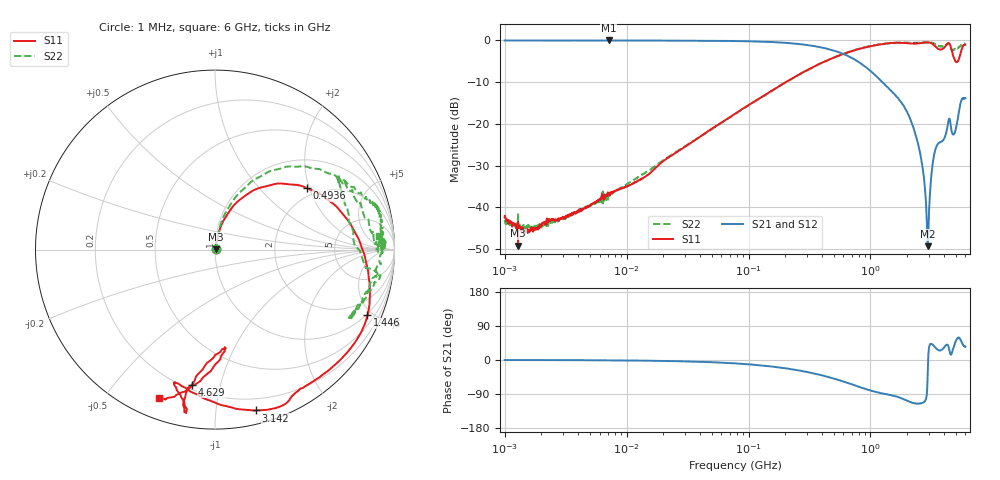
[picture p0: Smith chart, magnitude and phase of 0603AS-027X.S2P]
!s-Parameter Generated by FASTRON Sdn. Bhd.
!FASTRON P/N : 0603AS-027X
!Keysight Technologies: E5071C_MY46733604_B.14.02
!Date: Thu Nov 23 10:44:12 2023
!Version  :Rev01  Thu Nov 23 10:44:12 2023
!Data & Calibration Information:
!Freq  S11:SOLT2(ON)  S21:SOLT2(ON)  S12:SOLT2(ON)  S22:SOLT2(ON)
!PortZ  Port1:50+j0  Port2:50+j0
!When reading reference impedance value at option line is always used.
! Remarks : This data is being provided solely for informational purposes.
# Hz S dB R 50
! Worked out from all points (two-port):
!   1601 points, 1 MHz to 6 GHz, reference 50 ohm
!   highest |S21| = -0.04 dB at 7.15 MHz (marker M1); lowest = -49.3 dB at 2.951 GHz (marker M2)
!   |S21| within 3 dB of the highest: start of sweep to 570.2 MHz
!   lowest |S11| = -49.2 dB at 1.288 MHz (marker M3), VSWR 1.01, Z = 50.3 + j0.133 ohm
!   |S11| at or under -10 dB: start of sweep to 202.4 MHz
!   |S22| runs from -46.1 to -0.4 dB; largest |S21 - S12| = 0.0073
!   S11 on the Smith chart (normalised r, x): 1 MHz: 1.01, +0.01; 493.6 MHz: 1.74, +1.92; 1.446 GHz: 0.92, -4.68; 3.142 GHz: 0.10, -1.28; 4.629 GHz: 0.23, -0.82; 6 GHz: 0.09, -0.69
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1000000  -42.36 23.6  -0.04 -0.1  -0.05 -0.1  -43.05 22.6
1287650  -49.17 22.3  -0.05 -0.2  -0.02 -0.2  -41.46 12.8
4277066  -40.78 59.4  -0.06 -0.5  -0.05 -0.5  -40.67 59.7
7149933  -36.56 65.0  -0.04 -0.9  -0.06 -0.9  -37.04 74.5
1.823719e7  -29.93 77.7  -0.06 -2.2  -0.07 -2.2  -29.53 76.0
7.757876e7  -17.60 75.9  -0.17 -8.9  -0.18 -8.9  -17.66 77.6
3.307917e8  -6.56 49.6  -1.29 -34.3  -1.29 -34.3  -6.62 59.1
4.935518e8  -4.22 33.9  -2.41 -48.3  -2.41 -48.3  -4.21 48.8
8.659894e8  -1.84 2.7  -5.91 -74.0  -5.91 -74.1  -1.75 28.2
1.414819e9  -0.70 -22.3  -11.58 -92.0  -11.59 -92.0  -0.70 15.0
1.44567e9  -0.68 -23.3  -11.87 -92.2  -11.87 -92.2  -0.66 16.0
2.350488e9  -0.80 -59.2  -22.71 -114.6  -22.70 -114.5  -0.67 2.0
2.658144e9  -0.61 -63.5  -29.90 -113.5  -29.90 -113.4  -0.62 0.9
2.951149e9  -0.48 -68.2  -49.31 -27.5  -49.24 -27.3  -0.56 1.7
3.024401e9  -0.52 -70.6  -40.66 34.2  -40.63 34.1  -0.56 2.7
3.141603e9  -0.68 -75.7  -32.89 42.5  -32.87 42.4  -0.65 -0.9
3.42197e9  -1.55 -93.2  -25.92 31.8  -25.91 31.7  -1.07 -12.6
3.867453e9  -2.15 -106.8  -24.16 27.9  -24.18 27.8  -1.40 -26.1
4.312935e9  -0.73 -100.1  -20.06 38.8  -20.08 38.7  -0.75 -11.4
4.628987e9  -2.35 -99.7  -21.87 17.3  -21.90 17.2  -2.19 7.7
5.104645e9  -5.17 -84.4  -20.10 55.1  -20.11 55.2  -1.99 29.5
6e9  -1.07 -110.8  -13.90 34.9  -13.89 35.0  -0.73 4.7
